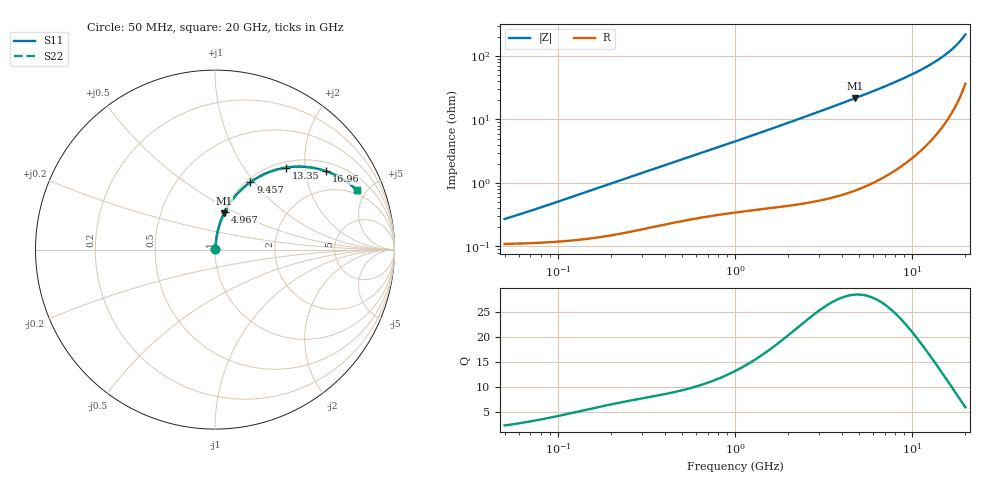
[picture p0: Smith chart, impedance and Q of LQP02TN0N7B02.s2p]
!Murata Part Number: LQP02TN0N7B02
!These Parameters are Measured in Series Mode Connection
!  o--[Z]--o
!Port1  Port2
!  o-------o
!Freq. Start=50[MHz] Stop=20[GHz], 401[Steps]
# Hz S RI R 50
!Freq.(Hz) S11(Real) S11(Imag) S21(Real) S21(Imag) S12(Real) S12(Imag) S22(Real) S22(Imag)
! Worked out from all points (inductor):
!   401 points, 50 MHz to 20 GHz, reference 50 ohm
!   read as one part in series: L = 787 pH near 68.48 MHz
!   highest Q = 28.5 at 4.748 GHz (marker M1), where L = 722 pH
!   S11 on the Smith chart (normalised r, x): 50 MHz: 1.00, +0.00; 4.967 GHz: 1.02, +0.45; 9.457 GHz: 1.04, +0.96; 13.35 GHz: 1.11, +1.59; 16.96 GHz: 1.27, +2.60; 20 GHz: 1.73, +4.31
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5e7  0.0011 0.00247  0.9989 -0.00247  0.9989 -0.00247  0.0011 0.00247
7.162978e7  0.00114 0.00354  0.9989 -0.00354  0.9989 -0.00354  0.00114 0.00354
1.364002e8  0.00133 0.00668  0.9987 -0.00668  0.9987 -0.00668  0.00133 0.00668
3.721004e8  0.00242 0.0175  0.9976 -0.0175  0.9976 -0.0175  0.00242 0.0175
1e9  0.00541 0.0446  0.9946 -0.0446  0.9946 -0.0446  0.00541 0.0446
1.714689e9  0.00981 0.0751  0.9902 -0.0751  0.9902 -0.0751  0.00981 0.0751
2.728004e9  0.0193 0.1183  0.9807 -0.1183  0.9807 -0.1183  0.0193 0.1183
3.626126e9  0.0311 0.1563  0.9689 -0.1563  0.9689 -0.1563  0.0311 0.1563
4.748272e9  0.0509 0.2028  0.9491 -0.2028  0.9491 -0.2028  0.0509 0.2028
4.966507e9  0.0553 0.2117  0.9447 -0.2117  0.9447 -0.2117  0.0553 0.2117
6.125241e9  0.0827 0.258  0.9173 -0.258  0.9173 -0.258  0.0827 0.258
7.442007e9  0.1215 0.3078  0.8785 -0.3078  0.8785 -0.3078  0.1215 0.3078
8.389408e9  0.1545 0.3412  0.8455 -0.3412  0.8455 -0.3412  0.1545 0.3412
9.457416e9  0.1969 0.3756  0.8031 -0.3756  0.8031 -0.3756  0.1969 0.3756
1.131968e10  0.284 0.4248  0.716 -0.4248  0.716 -0.4248  0.284 0.4248
1.238412e10  0.3407 0.4449  0.6593 -0.4449  0.6593 -0.4449  0.3407 0.4449
1.334722e10  0.3958 0.4569  0.6042 -0.4569  0.6042 -0.4569  0.3958 0.4569
1.527346e10  0.5134 0.46  0.4866 -0.46  0.4866 -0.46  0.5134 0.46
1.696185e10  0.619 0.4366  0.381 -0.4366  0.381 -0.4366  0.619 0.4366
1.828096e10  0.6982 0.4005  0.3018 -0.4005  0.3018 -0.4005  0.6982 0.4005
1.940974e10  0.7604 0.3576  0.2396 -0.3576  0.2396 -0.3576  0.7604 0.3576
2e10  0.79 0.3311  0.21 -0.3311  0.21 -0.3311  0.79 0.3311
